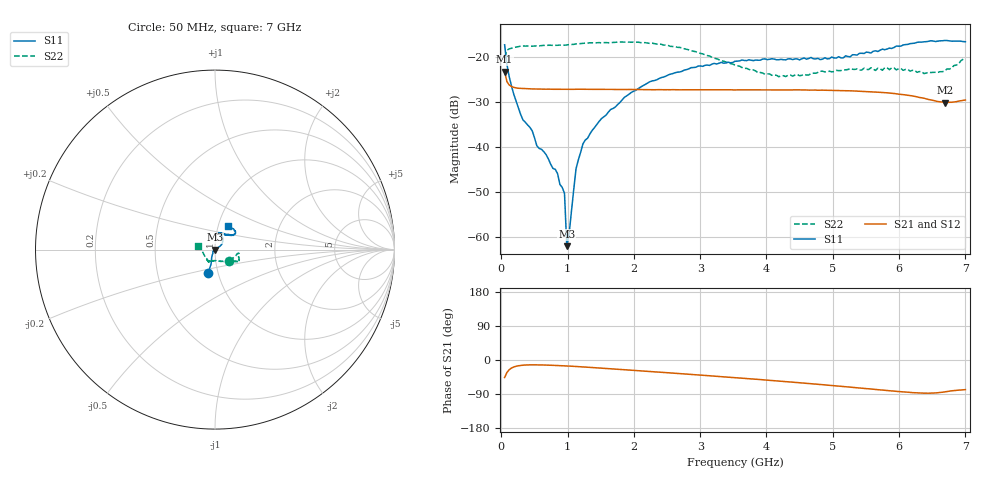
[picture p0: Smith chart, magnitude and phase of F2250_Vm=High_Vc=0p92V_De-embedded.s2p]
! Integrated Device Technology
! Corporate Headquarters
! 6024 Silver Creek Valley Road
! San Jose, CA 95138  USA
! Phone:  1-408-284-8200
! Toll Free:  1-800-223-1366
! Webpage:  http://www.idt.com/
! Timing and RF Division
! 515 Groton Road, Suite 102
! Westford, MA 01886-6024
! Device:  F2250
! Description: Voltage Variable RF Attenuator
! Frequency:  50.0 -  6000.00 MHz
! Package:  3x3 mm Thin QFN Plastic Package: 16 pin
! Ports:  2 RF, 3 DC
!  Pin  1  = GND
!  Pin  2  = NC
!  Pin  3  = RF1  = Port 1
!  Pin  4  = NC
!  Pin  5  = GND
!  Pin  6  = GND
!  Pin  7  = GND
!  Pin  8  = GND
!  Pin  9  = NC
!  Pin 10  = RF2  = Port 2
!  Pin 11  = NC
!  Pin 12  = GND
!  Pin 13  = GND
!  Pin 14  = VCNTRL
!  Pin 15  = VDD
!  Pin 16  = VMODE
! Vcntrl:  0.920 Volts
! Vmode:  +3.300 Volts
! Vdd:  +3.30  Volts
! Current:  1.317 mA
! Data:  The device was measured on a the F2250 evaluation board which has
!  individual transmission lines to the RF pins.  Data was collected
!  using a calibrated network analyzer.  The evaluation board was
!  de-embedded using a TRL calibration technique.
!  The reference plane is the edge of the package pin.
! Misc:  SN 10
!  Action Tracker AT0258
! Date Measured:  2014-11-26
! Date:  2015-10-15  MJV
! Note:
!  Integrated Device Technology supplies this data as a sample of measured
!  data at the package pin for this product.  Your particular data for this
!  product may vary.
!  Data was taken at 25 degrees C.
!  Integrated Device Technology reserves the right to change this data at anytime.
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# GHz S dB R 50
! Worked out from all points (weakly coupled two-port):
!   201 points, 50 MHz to 7 GHz, reference 50 ohm
!   highest |S21| = -23.16 dB at 50 MHz (marker M1); lowest = -30.1 dB at 6.687 GHz (marker M2)
!   lowest |S11| = -62.1 dB at 988.2 MHz (marker M3), VSWR 1.00, Z = 49.9 - j0.0121 ohm
!   |S11| at or under -10 dB: start of sweep to end of sweep
!   |S22| runs from -24.3 to -16.6 dB; largest |S21 - S12| = 0.00019
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0.05  -17.18 -106.8  -23.16 -46.2  -23.17 -46.2  -19.99 -38.0
0.08475  -21.51 -105.0  -25.39 -33.1  -25.38 -33.0  -18.40 -17.8
0.1195  -24.31 -108.9  -26.16 -25.6  -26.15 -25.6  -18.09 -12.0
0.29325  -32.78 -120.3  -26.91 -14.3  -26.90 -14.3  -17.46 -9.2
0.467  -36.40 -137.7  -27.03 -12.7  -27.03 -12.7  -17.50 -9.4
0.5365  -39.73 -143.9  -27.04 -12.8  -27.05 -12.8  -17.41 -10.7
0.8145  -44.98 173.4  -27.11 -14.3  -27.09 -14.3  -17.31 -15.0
0.9535  -50.36 -179.1  -27.11 -15.4  -27.12 -15.5  -17.27 -17.2
0.98825  -62.12 -171.1  -27.11 -15.8  -27.12 -15.8  -17.22 -17.6
1.023  -59.33 42.6  -27.13 -16.1  -27.13 -16.1  -17.14 -17.8
1.12725  -44.85 27.1  -27.10 -17.1  -27.10 -17.1  -16.99 -19.3
1.2315  -39.29 25.1  -27.09 -18.2  -27.09 -18.2  -16.84 -21.0
1.5095  -33.67 32.4  -27.13 -21.5  -27.12 -21.5  -16.74 -23.1
1.857  -28.90 34.5  -27.17 -25.7  -27.16 -25.7  -16.58 -25.6
2.37825  -24.73 43.6  -27.19 -32.0  -27.19 -32.0  -16.98 -28.7
2.86475  -22.27 55.1  -27.22 -38.1  -27.20 -38.2  -18.52 -33.1
3.525  -20.85 70.3  -27.26 -46.6  -27.26 -46.7  -21.71 -52.8
4.18525  -20.51 76.4  -27.24 -55.4  -27.26 -55.5  -24.30 -85.7
4.7065  -20.30 71.2  -27.28 -63.1  -27.29 -63.1  -23.52 -107.8
5.85325  -17.93 39.8  -27.96 -81.0  -27.95 -81.2  -22.73 -119.6
6.68725  -16.23 47.2  -30.07 -84.1  -30.10 -84.2  -23.03 -171.1
7  -16.50 61.9  -29.49 -78.1  -29.50 -78.2  -20.18 166.9
